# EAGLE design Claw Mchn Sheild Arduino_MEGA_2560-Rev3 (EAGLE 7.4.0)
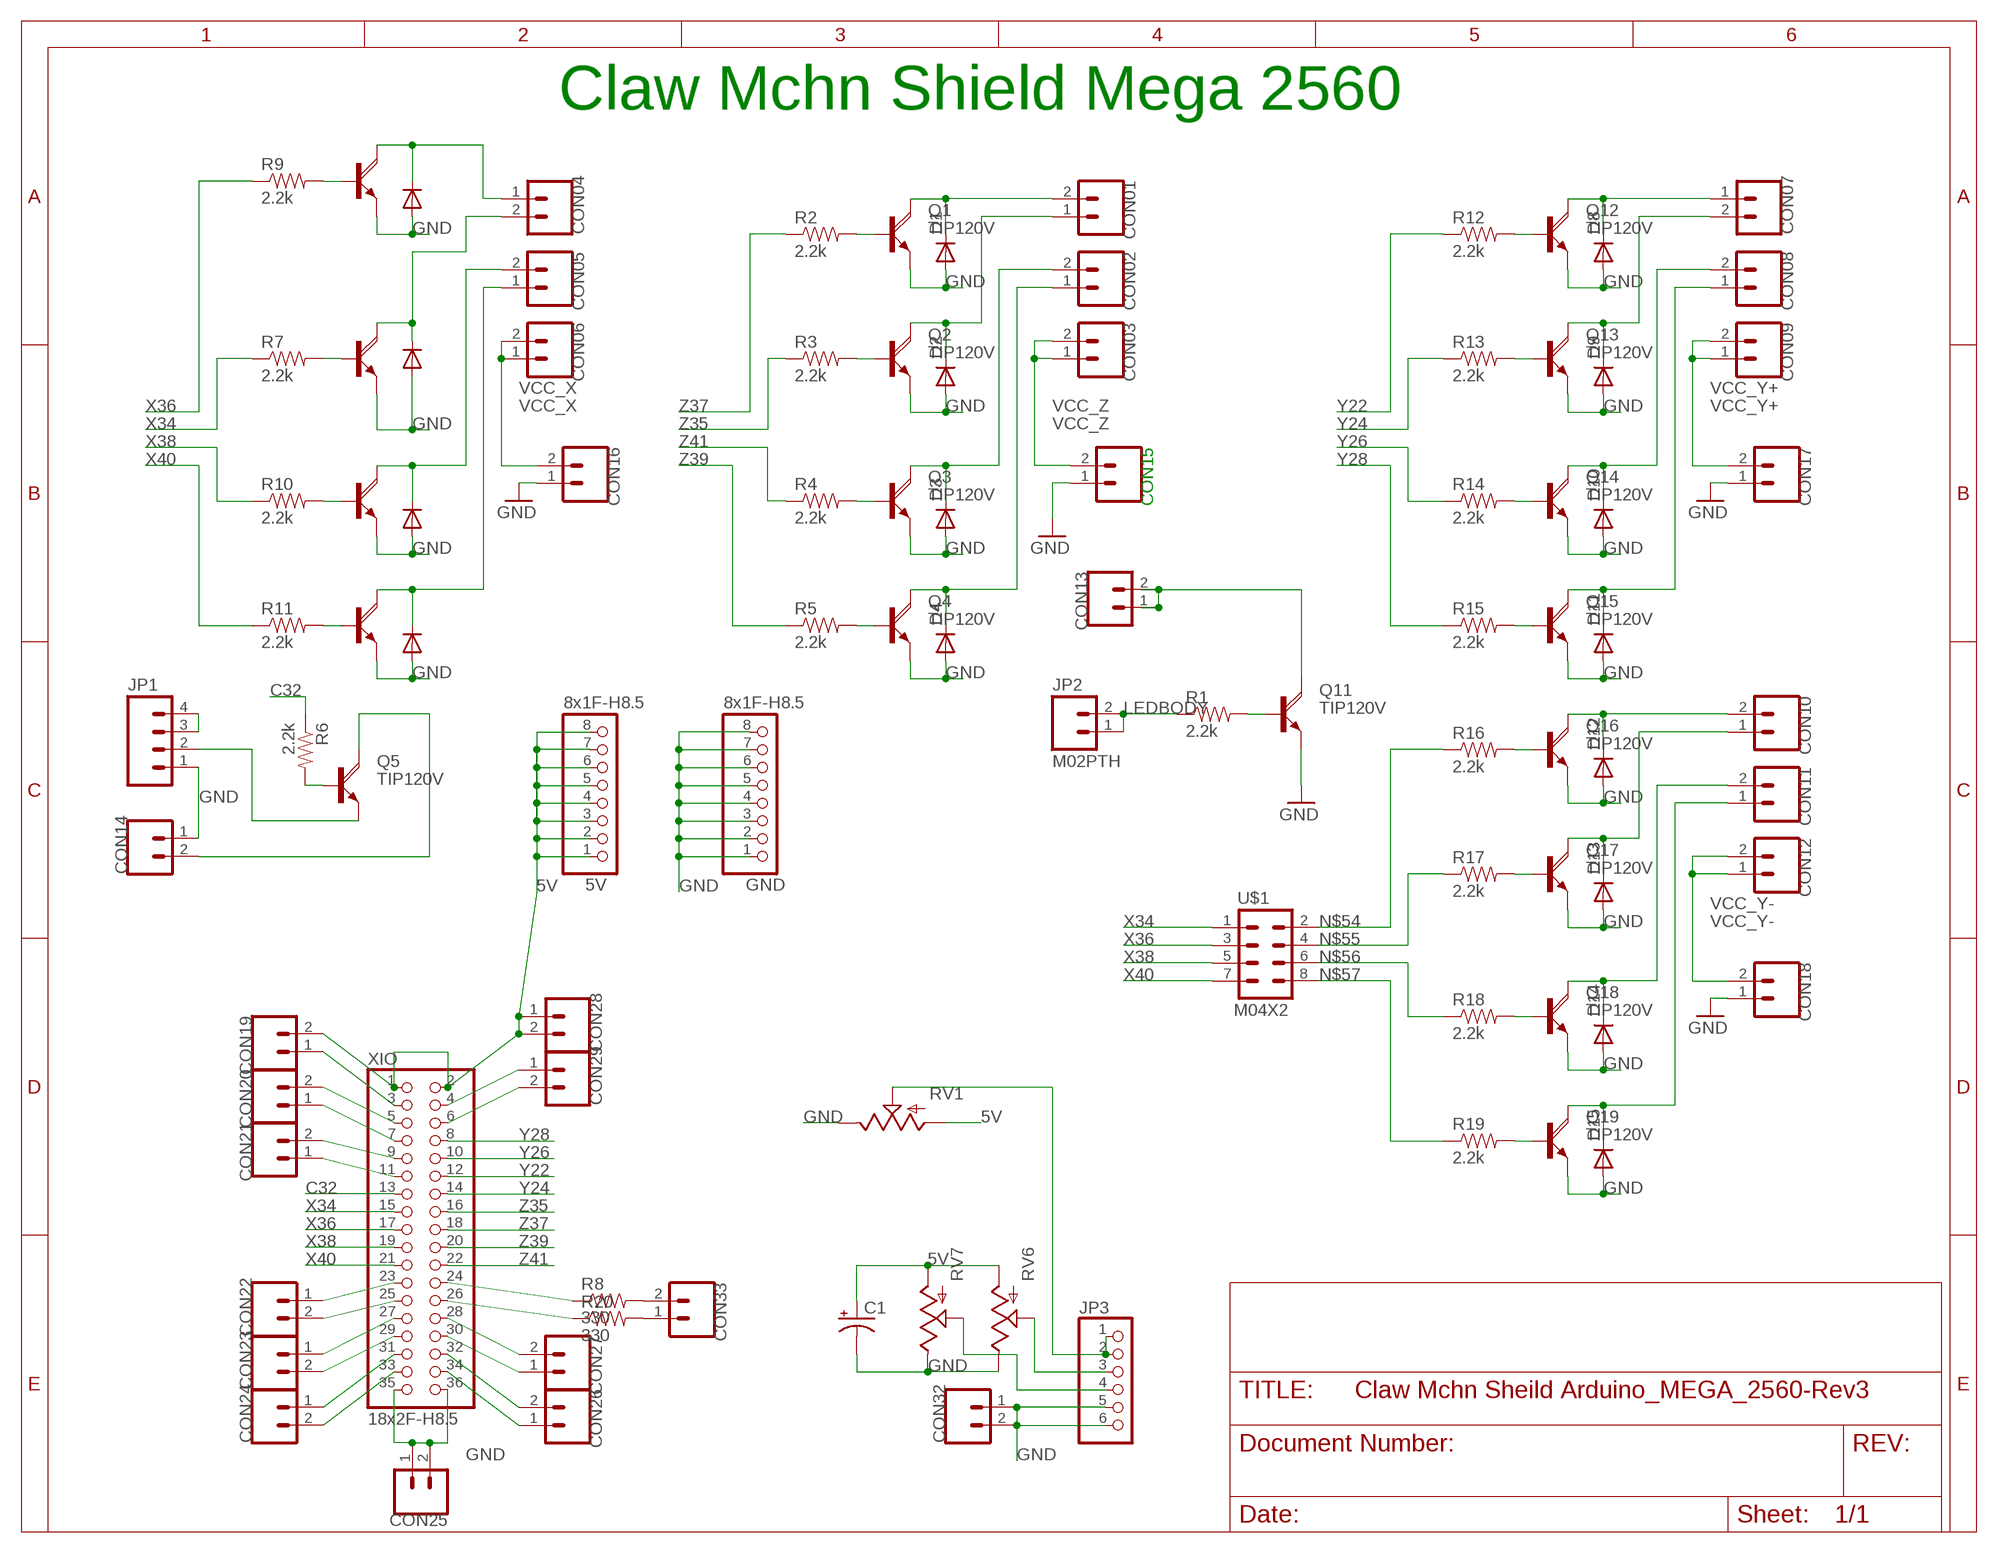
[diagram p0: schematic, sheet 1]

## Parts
5V  8x1F-H8.5  PINHD-1X8  [1X08]
C1  CAP_POLPTH1  [CPOL-RADIAL-100UF-25V]
CON01  M023.5MM  [SCREWTERMINAL-3.5MM-2]
CON02  M023.5MM  [SCREWTERMINAL-3.5MM-2]
CON03  M023.5MM  [SCREWTERMINAL-3.5MM-2]
CON04  M023.5MM  [SCREWTERMINAL-3.5MM-2]
CON05  M023.5MM  [SCREWTERMINAL-3.5MM-2]
CON06  M023.5MM  [SCREWTERMINAL-3.5MM-2]
CON07  M023.5MM  [SCREWTERMINAL-3.5MM-2]
CON08  M023.5MM  [SCREWTERMINAL-3.5MM-2]
CON09  M023.5MM  [SCREWTERMINAL-3.5MM-2]
CON10  M023.5MM  [SCREWTERMINAL-3.5MM-2]
CON11  M023.5MM  [SCREWTERMINAL-3.5MM-2]
CON12  M023.5MM  [SCREWTERMINAL-3.5MM-2]
CON13  M023.5MM  [SCREWTERMINAL-3.5MM-2]
CON14  M023.5MM  [SCREWTERMINAL-3.5MM-2]
CON15  M023.5MM  [SCREWTERMINAL-3.5MM-2]
CON16  M023.5MM  [SCREWTERMINAL-3.5MM-2]
CON17  M023.5MM  [SCREWTERMINAL-3.5MM-2]
CON18  M023.5MM  [SCREWTERMINAL-3.5MM-2]
CON19  M023.5MM  [SCREWTERMINAL-3.5MM-2]
CON20  M023.5MM  [SCREWTERMINAL-3.5MM-2]
CON21  M023.5MM  [SCREWTERMINAL-3.5MM-2]
CON22  M023.5MM  [SCREWTERMINAL-3.5MM-2]
CON23  M023.5MM  [SCREWTERMINAL-3.5MM-2]
CON24  M023.5MM  [SCREWTERMINAL-3.5MM-2]
CON25  M023.5MM  [SCREWTERMINAL-3.5MM-2]
CON26  M023.5MM  [SCREWTERMINAL-3.5MM-2]
CON27  M023.5MM  [SCREWTERMINAL-3.5MM-2]
CON28  M023.5MM  [SCREWTERMINAL-3.5MM-2]
CON29  M023.5MM  [SCREWTERMINAL-3.5MM-2]
CON32  M023.5MM  [SCREWTERMINAL-3.5MM-2]
CON33  M023.5MM  [SCREWTERMINAL-3.5MM-2]
D1  DIODE-SOT54H  [SOT54H]
D2  DIODE-SOT54H  [SOT54H]
D3  DIODE-SOT54H  [SOT54H]
D4  DIODE-SOT54H  [SOT54H]
D5  DIODE-SOT54H  [SOT54H]
D6  DIODE-SOT54H  [SOT54H]
D7  DIODE-SOT54H  [SOT54H]
D8  DIODE-SOT54H  [SOT54H]
D9  DIODE-SOT54H  [SOT54H]
D10  DIODE-SOT54H  [SOT54H]
D11  DIODE-SOT54H  [SOT54H]
D12  DIODE-SOT54H  [SOT54H]
D13  DIODE-SOT54H  [SOT54H]
D14  DIODE-SOT54H  [SOT54H]
D15  DIODE-SOT54H  [SOT54H]
D16  DIODE-SOT54H  [SOT54H]
GND  8x1F-H8.5  PINHD-1X8  [1X08]
JP1  M04PTH  [1X04]
JP2  M02PTH  [1X02]
JP3  PINHD-1X6  [1X06]
Q1  TIP120V  [TO220AV]
Q2  TIP120V  [TO220AV]
Q3  TIP120V  [TO220AV]
Q4  TIP120V  [TO220AV]
Q5  TIP120V  [TO220AV]
Q6  TIP120V  [TO220AV]
Q8  TIP120V  [TO220AV]
Q9  TIP120V  [TO220AV]
Q10  TIP120V  [TO220AV]
Q11  TIP120V  [TO220AV]
Q12  TIP120V  [TO220AV]
Q13  TIP120V  [TO220AV]
Q14  TIP120V  [TO220AV]
Q15  TIP120V  [TO220AV]
Q16  TIP120V  [TO220AV]
Q17  TIP120V  [TO220AV]
Q18  TIP120V  [TO220AV]
Q19  TIP120V  [TO220AV]
R1  2.2k  RESISTORPTH-1/6W  [1/6W-RES]
R2  2.2k  RESISTORPTH-1/6W  [1/6W-RES]
R3  2.2k  RESISTORPTH-1/6W  [1/6W-RES]
R4  2.2k  RESISTORPTH-1/6W  [1/6W-RES]
R5  2.2k  RESISTORPTH-1/6W  [1/6W-RES]
R6  2.2k  RESISTORPTH-1/6W  [1/6W-RES]
R7  2.2k  RESISTORPTH-1/6W  [1/6W-RES]
R8  330  RESISTORPTH-1/4W  [AXIAL-0.4]
R9  2.2k  RESISTORPTH-1/6W  [1/6W-RES]
R10  2.2k  RESISTORPTH-1/6W  [1/6W-RES]
R11  2.2k  RESISTORPTH-1/6W  [1/6W-RES]
R12  2.2k  RESISTORPTH-1/6W  [1/6W-RES]
R13  2.2k  RESISTORPTH-1/6W  [1/6W-RES]
R14  2.2k  RESISTORPTH-1/6W  [1/6W-RES]
R15  2.2k  RESISTORPTH-1/6W  [1/6W-RES]
R16  2.2k  RESISTORPTH-1/6W  [1/6W-RES]
R17  2.2k  RESISTORPTH-1/6W  [1/6W-RES]
R18  2.2k  RESISTORPTH-1/6W  [1/6W-RES]
R19  2.2k  RESISTORPTH-1/6W  [1/6W-RES]
R20  330  RESISTORPTH-1/4W  [AXIAL-0.4]
RV1  POTTRIM  [TRIM_POT]
RV6  POTTRIM  [TRIM_POT]
RV7  POTTRIM  [TRIM_POT]
U$1  M04X2  [2X4]
XIO  18x2F-H8.5  PINHD-2X18  [2X18]

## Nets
5V: 5V.1 5V.2 5V.3 5V.4 5V.5 5V.6 5V.7 5V.8 C1.1(+) CON19.2 CON28.1 CON28.2 RV1.3(A) RV6.3(A) RV7.3(A) XIO.1 XIO.2
C32: R6.1 XIO.13
GND: C1.2(-) CON14.1 CON15.1 CON16.1 CON17.1 CON18.1 CON25.1 CON25.2 CON32.1 CON32.2 D1.A D2.A D3.A D4.A D5.A D6.A D7.A D8.A D9.A D10.A D11.A D12.A D13.A D14.A D15.A D16.A GND.1 GND.2 GND.3 GND.4 GND.5 GND.6 GND.7 GND.8 JP1.1 JP3.5 JP3.6 Q1.E Q2.E Q3.E Q4.E Q6.E Q8.E Q9.E Q10.E Q11.E Q12.E Q13.E Q14.E Q15.E Q16.E Q17.E Q18.E Q19.E RV1.2(E) RV6.2(E) RV7.2(E) XIO.35 XIO.36
LEDBODY: JP2.1 JP2.2 R1.1
N$1: Q11.B R1.2
N$2: Q1.B R2.2
N$3: Q2.B R3.2
N$4: Q3.B R4.2
N$5: Q4.B R5.2
N$6: CON33.1 R20.P$2
N$7: CON04.2 D16.C Q6.C
N$8: CON26.1 XIO.34
N$9: CON27.1 XIO.30
N$10: CON01.2 D1.C Q1.C
N$11: CON01.1 D2.C Q2.C
N$12: CON02.2 D3.C Q3.C
N$13: CON02.1 D4.C Q4.C
N$14: CON21.1 XIO.11
N$15: CON33.2 R8.P$2
N$16: JP1.2 Q5.E
N$17: Q6.B R7.2
N$18: Q5.B R6.2
N$19: JP3.4 RV7.1(S)
N$21: CON29.1 XIO.4
N$22: R20.P$1 XIO.26
N$23: CON14.2 Q5.C
N$24: R8.P$1 XIO.24
N$25: Q8.B R9.2
N$26: Q9.B R10.2
N$27: Q10.B R11.2
N$28: CON21.2 XIO.9
N$29: CON26.2 XIO.32
N$30: CON27.2 XIO.28
N$31: CON20.1 XIO.7
N$32: CON20.2 XIO.5
N$33: CON04.1 D5.C Q8.C
N$34: CON05.2 D6.C Q9.C
N$35: CON05.1 D7.C Q10.C
N$36: Q12.B R12.2
N$37: CON24.2 XIO.33
N$38: Q13.B R13.2
N$39: CON13.1 CON13.2 Q11.C
N$40: Q14.B R14.2
N$41: Q15.B R15.2
N$42: CON24.1 XIO.31
N$43: CON23.2 XIO.29
N$44: CON23.1 XIO.27
N$45: CON22.2 XIO.25
N$46: CON07.1 D8.C Q12.C
N$47: CON07.2 D9.C Q13.C
N$48: CON08.2 D10.C Q14.C
N$49: CON08.1 D11.C Q15.C
N$50: Q16.B R16.2
N$51: Q17.B R17.2
N$52: Q18.B R18.2
N$53: Q19.B R19.2
N$54: R16.1 U$1.2
N$55: R17.1 U$1.4
N$56: R18.1 U$1.6
N$57: R19.1 U$1.8
N$58: CON10.2 D12.C Q16.C
N$59: CON10.1 D13.C Q17.C
N$60: CON11.2 D14.C Q18.C
N$61: CON11.1 D15.C Q19.C
N$62: CON19.1 XIO.3
N$63: CON22.1 XIO.23
N$65: JP1.3 JP1.4
N$66: CON29.2 XIO.6
N$67: JP3.3 RV6.1(S)
N$74: JP3.1 JP3.2 RV1.1(S)
VCC_X: CON06.1 CON06.2 CON16.2
VCC_Y+: CON09.1 CON09.2 CON17.2
VCC_Y-: CON12.1 CON12.2 CON18.2
VCC_Z: CON03.1 CON03.2 CON15.2
X34: R7.1 U$1.1 XIO.15
X36: R9.1 U$1.3 XIO.17
X38: R10.1 U$1.5 XIO.19
X40: R11.1 U$1.7 XIO.21
Y22: R12.1 XIO.12
Y24: R13.1 XIO.14
Y26: R14.1 XIO.10
Y28: R15.1 XIO.8
Z35: R3.1 XIO.16
Z37: R2.1 XIO.18
Z39: R5.1 XIO.20
Z41: R4.1 XIO.22

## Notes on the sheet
- Claw Mchn Shield Mega 2560

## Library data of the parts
5V GND = SmartPrj:PINHD-1X8: PIN HEADER
C1 = SparkFun-Capacitors:CAP_POL: Capacitor Polarized
CON01-CON09 CON10-CON29 CON32 CON33 JP2 = SparkFun-Connectors:M02: Standard 2-pin 0.1" header. Use with
D1-D16 = diode:DIODE-: DIODE
JP1 = SparkFun-Connectors:M04: Header 4 Standard 4-pin 0.1" header. Use with straight break away headers (SKU : PRT-00116), right angle break away headers (PRT-00553), swiss pins (PRT-00743), machine pins (PRT-00117), and female headers (PRT-00115). Molex polarized connector foot print use with SKU : PRT-08231 with associated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
JP3 = pinhead:PINHD-1X6: PIN HEADER
Q1-Q6 Q8-Q19 = rocketfarm:TIP120: NPN DARLINGTON TRANSISTOR
R1-R20 = SparkFun-Passives:RESISTOR: Resistor
RV1 RV6 RV7 = SparkFun-Electromechanical:POT
U$1 = SparkFun-Connectors:M04X2: .1" header, two rows of four.
XIO = SmartPrj:PINHD-2X18: PIN HEADER

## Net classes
1 power: width 0.61 mm, drill 0.406 mm, clearance 0.203 mm
2 gnd: width 0.305 mm, drill 0.406 mm, clearance 0.203 mm
3 power usb: width 0.508 mm, drill 0.406 mm, clearance 0.203 mm

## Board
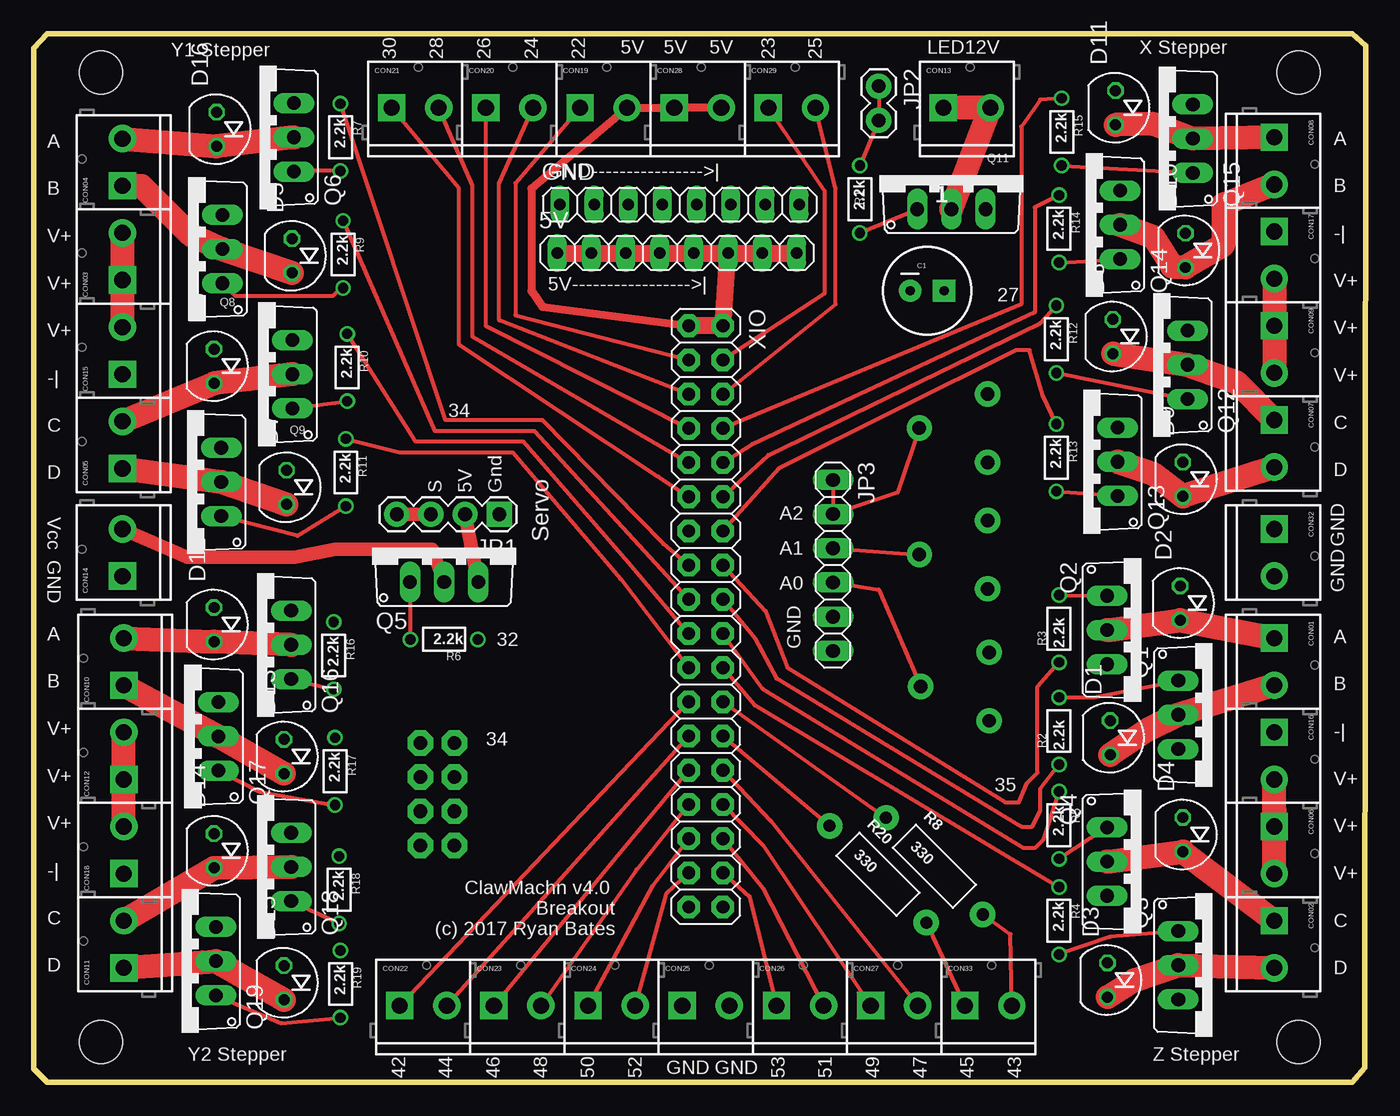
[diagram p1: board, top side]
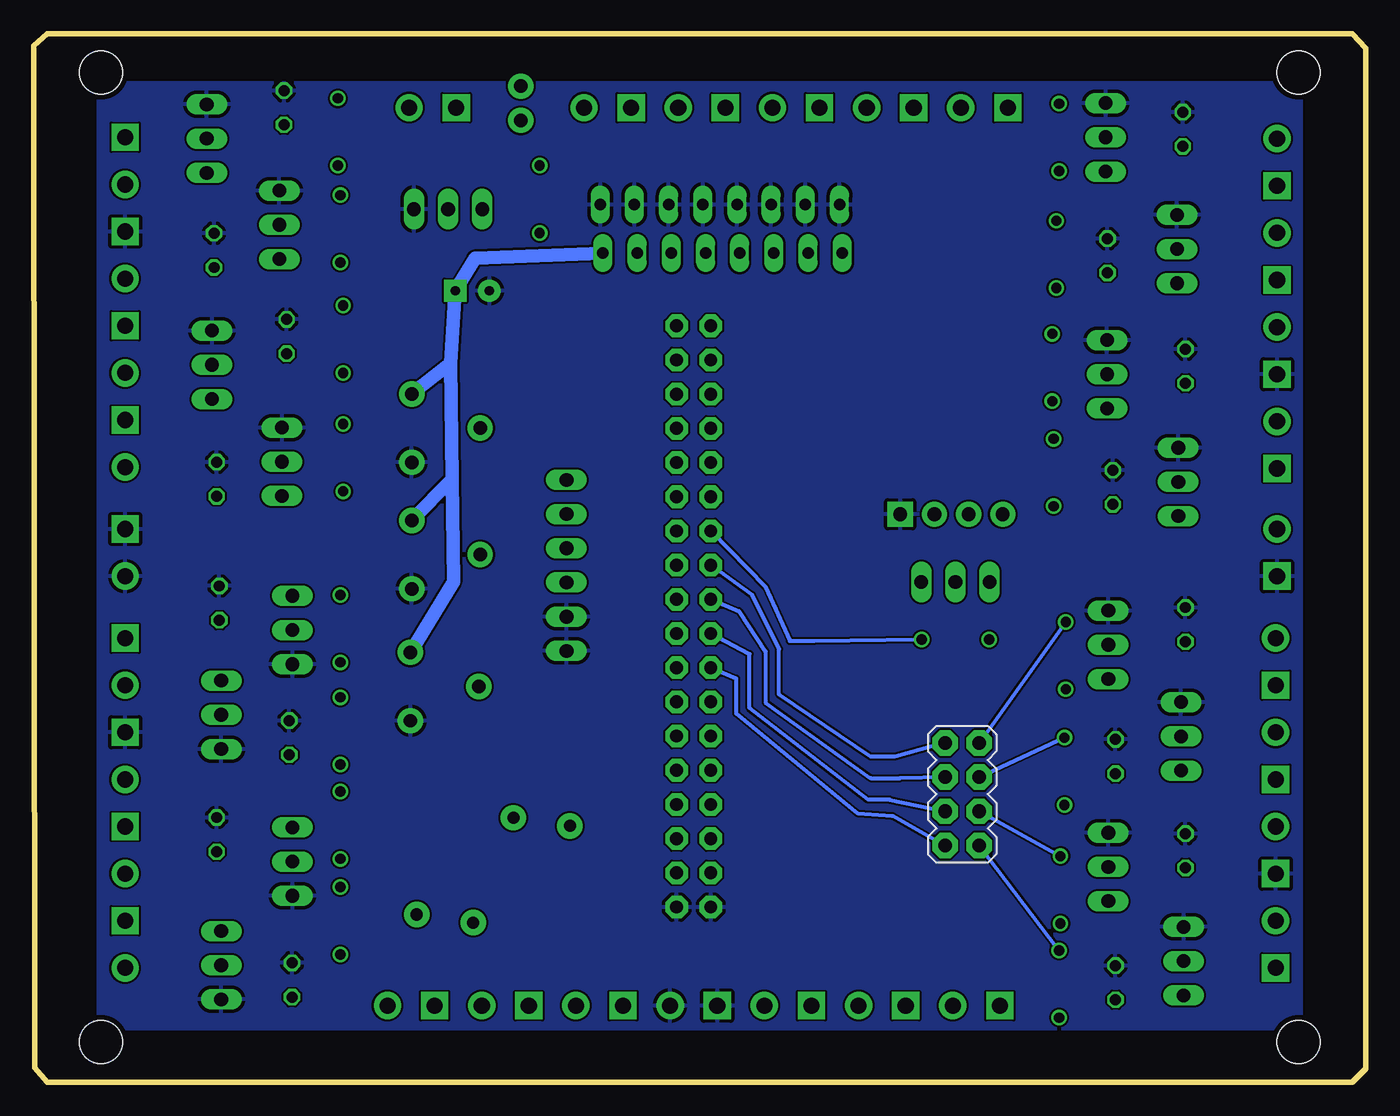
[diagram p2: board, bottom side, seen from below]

Size 99 x 77.9 mm. Coordinates in mm from the lower left corner, seen from the top.
Outline: 1,77.9 98,77.9 99,77 98.9,1.1 98,0 1,0 0,1 0,76.8 1,77.9
Copper layers (1*16): Top 0.0356mm / dielectric 1.5011mm / Bottom 0.0356mm
Design rules "OSHparkPCBOrder": minimum track width 6mil, minimum drill 13mil, track to track 6mil, track to pad 6mil, pad to pad 6mil, via to via 6mil, smd to smd 6mil, copper to edge 15mil, drill to drill 6mil, minimum pad ring 7mil, minimum via ring 7mil, stop-mask expansion 3mil, vias tented up to drill 0mil, thermal gap 10mil
Holes 3.2 mm at 94,3 5,75 94,75 5,3

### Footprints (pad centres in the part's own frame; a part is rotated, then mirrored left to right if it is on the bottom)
1X08 = drill 0.85 pad 1.422 long: 1 -8.89,0; 2 -6.35,0; 3 -3.81,0; 4 -1.27,0; 5 1.27,0; 6 3.81,0; 7 6.35,0; 8 8.89,0
CPOL-RADIAL-100UF-25V = drill 0.7 pad 1.651 square: 1 1.27,0 | drill 0.7 pad 1.651: 2 -1.27,0
SCREWTERMINAL-3.5MM-2 = drill 1.2 pad 2.032 square: 1 0,0 | drill 1.2 pad 2.032: 2 3.5,0
SOT54H = drill 0.813 octagon: A 1.27,0; C -1.27,0
1X04 = drill 1.016 pad 1.88 square: 1 0,0 | drill 1.016 pad 1.88: 2 2.54,0; 3 5.08,0; 4 7.62,0
1X02 = drill 1.016 pad 1.88: 1 0,0; 2 2.54,0
1X06 = drill 1.016 long: 1 -6.35,0; 2 -3.81,0; 3 -1.27,0; 4 1.27,0; 5 3.81,0; 6 6.35,0
TO220AV = drill 1.016 long: B -2.54,-2.54; C 0,-2.54; E 2.54,-2.54
1/6W-RES = drill 0.762: 1 -2.5,0; 2 2.5,0
AXIAL-0.4 = drill 0.9 pad 1.88: P$1 -5.08,0; P$2 5.08,0
TRIM_POT = drill 1 pad 1.88: 1 5.08,0; 2 0,2.54; 3 0,-2.54
2X4 = drill 1.016 pad 1.88 octagon: 1 -3.81,-1.27; 2 -3.81,1.27; 3 -1.27,-1.27; 4 -1.27,1.27; 5 1.27,-1.27; 6 1.27,1.27; 7 3.81,-1.27; 8 3.81,1.27
2X18 = drill 0.95 pad 1.676 octagon: 1 -21.59,-1.27; 2 -21.59,1.27; 3 -19.05,-1.27; 4 -19.05,1.27; 5 -16.51,-1.27; 6 -16.51,1.27; 7 -13.97,-1.27; 8 -13.97,1.27; 9 -11.43,-1.27; 10 -11.43,1.27; 11 -8.89,-1.27; 12 -8.89,1.27; 13 -6.35,-1.27; 14 -6.35,1.27; 15 -3.81,-1.27; 16 -3.81,1.27; 17 -1.27,-1.27; 18 -1.27,1.27; 19 1.27,-1.27; 20 1.27,1.27; 21 3.81,-1.27; 22 3.81,1.27; 23 6.35,-1.27; 24 6.35,1.27; 25 8.89,-1.27; 26 8.89,1.27; 27 11.43,-1.27; 28 11.43,1.27; 29 13.97,-1.27; 30 13.97,1.27; 31 16.51,-1.27; 32 16.51,1.27; 33 19.05,-1.27; 34 19.05,1.27; 35 21.59,-1.27; 36 21.59,1.27

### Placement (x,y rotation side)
5V  47.8,61.6 0 top
C1  66.4,58.8 0 top
CON01  92.2,33 270 top
CON02  92.2,12 270 top
CON03  6.6,59.6 90 top
CON04  6.6,66.6 90 top
CON05  6.6,45.6 90 top
CON06  92.2,19 270 top
CON07  92.2,49.2 270 top
CON08  92.2,70.2 270 top
CON09  92.2,56.2 270 top
CON10  6.7,29.5 90 top
CON11  6.7,8.5 90 top
CON12  6.7,22.5 90 top
CON13  67.6,72.4 0 top
CON14  6.6,37.6 90 top
CON15  6.6,52.6 90 top
CON16  92.2,26 270 top
CON17  92.2,63.2 270 top
CON18  6.7,15.5 90 top
CON19  40.6,72.4 0 top
CON20  33.6,72.4 0 top
CON21  26.6,72.4 0 top
CON22  27.2,5.7 0 top
CON23  34.2,5.7 0 top
CON24  41.2,5.7 0 top
CON25  48.2,5.7 0 top
CON26  55.2,5.7 0 top
CON27  62.2,5.7 0 top
CON28  47.6,72.4 0 top
CON29  54.6,72.4 0 top
CON32  92.2,41.1 270 top
CON33  69.2,5.7 0 top
D1  80,25.6 90 top
D2  85.2,35.6 90 top
D3  79.8,7.6 90 top
D4  85.4,18.4 90 top
D5  19.2,61.4 90 top
D6  13.4,53.2 90 top
D7  18.8,44.2 90 top
D8  80.2,55.4 90 top
D9  85.4,44.8 90 top
D10  85.6,61.8 90 top
D11  80.4,72.4 90 top
D12  13.4,34 90 top
D13  18.6,24.2 90 top
D14  13.4,17.2 90 top
D15  18.6,7.4 90 top
D16  13.6,70.8 90 top
GND  48,65.2 0 top
JP1  34.6,42.2 180 top
JP2  62.8,74 270 top
JP3  59.4,38.4 270 top
Q1  87.6,27.3 270 top
Q2  82.3,33.6 270 top
Q3  87.6,8.7 270 top
Q4  82.3,16.4 270 top
Q5  30.5,39.7 0 top
Q6  16.8,70.2 90 top
Q8  11.5,61.9 90 top
Q9  16.7,52.6 90 top
Q10  11.4,44.6 90 top
Q11  68.2,67.4 0 top
Q12  83.2,53.3 90 top
Q13  78,46.1 90 top
Q14  78.2,63.7 90 top
Q15  83.6,70.1 90 top
Q16  16.6,32.5 90 top
Q17  11.2,25.7 90 top
Q18  16.6,16 90 top
Q19  11,9 90 top
R1  61.4,65.6 270 top
R2  76.2,26.1 90 top
R3  76.2,33.7 90 top
R4  76.2,12 270 top
R5  76.2,19.1 270 top
R6  30.5,32.9 180 top
R7  22.8,70.2 270 top
R8  66.94,16.06 315 top
R9  23,61.5 270 top
R10  23.3,53.1 270 top
R11  23.2,45.3 270 top
R12  76,55.2 270 top
R13  76,46.4 270 top
R14  76.2,63.4 270 top
R15  76.4,70.6 270 top
R16  22.3,31.7 270 top
R17  22.4,23.1 270 top
R18  22.7,14.3 270 top
R19  22.8,7.3 270 top
R20  62.74,15.46 315 top
RV1  70.9,48.6 180 top
RV6  70.9,39.2 180 top
RV7  71,29.4 180 top
U$1  30,21.4 270 bottom
XIO  49.95,34.61 270 top

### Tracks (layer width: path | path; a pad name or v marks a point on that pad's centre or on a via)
5V
  Top 0.61: CON28.2 CON28.1 CON19.2 37,66.4 37,58.8 37.8,57.6 XIO.1
  Top 1.27: XIO.1 XIO.2 5V.6 | 5V.1 5V.2 5V.3 5V.4 5V.5 5V.6 | 5V.6 5V.7 5V.8
  Bottom 1.016: 5V.8 66.2,61.2 C1.1 68.01,53.4 | 68.01,53.4 67.9,44.81 | 67.9,44.81 67.8,37.2 RV7.3 | RV6.3 67.9,44.81 | RV1.3 68.01,53.4
C32
  Bottom 0.305: XIO.13 44.6,36.8 42.8,32.8 41,32.8 R6.1
GND
  pour Bottom: 4.8,74.2 94.2,74.2 94.2,4 4.8,4
LEDBODY
  Top 0.305: JP2.1 JP2.2 R1.1
N$1
  Top 0.305: R1.2 Q11.B
N$2
  Top 0.305: R2.2 78.8,28.6 Q1.B
N$3
  Top 0.305: R3.2 Q2.B
N$4
  Top 0.305: Q3.B 80,10.8 R4.2
N$5
  Top 0.305: R5.2 Q4.B
N$6
  Top 0.305: R20.P$2 CON33.1
N$7
  Top 1.778: CON04.2 D16.C Q6.C
N$8
  Top 0.305: XIO.34 53.2,13.8 CON26.1
N$9
  Top 0.305: XIO.30 54.2,17.6 CON27.1
N$10
  Top 1.778: CON01.2 Q1.C 82.8,26.2 D1.C
N$11
  Top 1.778: Q2.C D2.C CON01.1
N$12
  Top 1.778: CON02.2 Q3.C 81.8,7.6 D3.C
N$13
  Top 1.778: Q4.C D4.C CON02.1
N$14
  Top 0.305: XIO.11 46.4,45 31.6,54.8 31.6,66.4 CON21.1
N$15
  Top 0.305: CON33.2 72.6,11 R8.P$2
N$16
  Top 1.016: JP1.2 Q5.E
N$17
  Top 0.305: R7.2 19.38,67.7 Q6.B
N$18
  Top 0.305: R6.2 28,34.4 Q5.B
N$19
  Top 0.305: JP3.4 62.8,36.6 RV7.1
N$21
  Top 0.305: XIO.4 58.8,58.6 58.8,66.2 CON29.1
N$22
  Top 0.305: R20.P$1 XIO.26
N$23
  Top 1.016: Q5.C 29.6,39.6 22.4,39.6 19.4,39 11.4,39 CON14.2
N$24
  Top 0.305: XIO.24 R8.P$1
N$25
  Top 0.305: R9.2 22.8,59 22.2,58.4 15,58.4 Q8.B
N$26
  Top 0.305: Q9.B R10.2
N$27
  Top 0.305: R11.2 19.6,40.6 Q10.B
N$28
  Top 0.305: XIO.9 32.6,55.4 32.6,66.6 CON21.2
N$29
  Top 0.305: XIO.32 54.2,14.4 CON26.2
N$30
  Top 0.305: XIO.28 54.8,19.4 CON27.2
N$31
  Top 0.305: CON20.1 33.6,56.2 XIO.7
N$32
  Top 0.305: XIO.5 34.6,56.6 34.6,66.8 CON20.2
N$33
  Top 1.778: CON04.1 8,66.6 11.6,63 Q8.C D5.C
N$34
  Top 1.778: Q9.C D6.C CON05.2
N$35
  Top 1.778: CON05.1 Q10.C D7.C
N$36
  Top 0.305: R12.2 Q12.B
N$37
  Top 0.305: XIO.33 47,14 CON24.2
N$38
  Top 0.305: R13.2 Q13.B
N$39
  Top 1.778: Q11.C CON13.2 CON13.1
N$40
  Top 0.305: R14.2 Q14.B
N$41
  Top 0.305: R15.2 Q15.B
N$42
  Top 0.305: XIO.31 46,14.6 CON24.1
N$43
  Top 0.305: XIO.29 44.8,15.8 CON23.2
N$44
  Top 0.305: XIO.27 43.2,16.6 CON23.1
N$45
  Top 0.305: XIO.25 CON22.2
N$46
  Top 1.778: D8.C Q12.C 89.4,52 CON07.1
N$47
  Top 1.778: CON07.2 D9.C 83.2,45.2 Q13.C
N$48
  Top 1.778: Q14.C 83.2,62.8 84.6,60.6 D10.C 88.4,62.2 88.4,65.2 CON08.2
N$49
  Top 1.778: CON08.1 Q15.C 83.2,71.2 D11.C
N$50
  Top 0.305: Q16.B R16.2
N$51
  Top 0.305: Q17.B 16.8,21.6 R17.2
N$52
  Top 0.305: Q18.B R18.2
N$53
  Top 0.305: Q19.B 18.4,4.4 R19.2
N$54
  Bottom 0.305: R16.1 U$1.2
N$55
  Bottom 0.305: R17.1 U$1.4
N$56
  Bottom 0.305: R18.1 U$1.6
N$57
  Bottom 0.305: R19.1 U$1.8
N$58
  Top 1.778: CON10.2 D12.C Q16.C
N$59
  Top 1.778: CON10.1 Q17.C D13.C
N$60
  Top 1.778: CON11.2 D14.C Q18.C
N$61
  Top 1.778: CON11.1 Q19.C D15.C
N$62
  Top 0.305: CON19.1 35.8,66.8 35.8,57 XIO.3
N$63
  Top 0.305: XIO.23 CON22.1
N$65
  Top 1.016: JP1.4 JP1.3
N$66
  Top 0.305: XIO.6 59.6,57.8 59.6,66.4 CON29.2
N$67
  Top 0.305: JP3.3 RV6.1
N$74
  Top 0.305: RV1.1 64.2,43.8 JP3.2 JP3.1
VCC_X
  Top 1.778: CON16.2 92.2,20.2 CON06.1 CON06.2
VCC_Y+
  Top 1.778: CON17.2 CON09.1 CON09.2
VCC_Y-
  Top 1.778: CON18.2 CON12.1 CON12.2
VCC_Z
  Top 1.778: CON15.2 CON03.1 CON03.2
X34
  Top 0.305: XIO.15 46.8,40 37.8,49.2 30.6,49.2 R7.1
  Bottom 0.305: XIO.15 45.6,36.2 43.6,32.2 43.6,28.8 36.8,24.2 35,24.2 U$1.1
X36
  Top 0.305: R9.1 29.8,48.4 37.2,48.4 XIO.17
  Bottom 0.305: XIO.17 46.6,35 44.6,32 44.6,28.2 36.8,22.6 34.6,22.6 U$1.3
X38
  Top 0.305: XIO.19 44.2,38.6 36.4,47.6 28.4,47.6 R10.1
  Bottom 0.305: XIO.19 45.8,31.8 45.8,27.8 37,21 35.4,21 U$1.5
X40
  Top 0.305: R11.1 27.2,46.8 35.6,46.8 43.6,37.4 XIO.21
  Bottom 0.305: XIO.21 46.8,30 46.8,27.4 37.8,20 35.2,19.8 U$1.7
Y22
  Top 0.305: XIO.12 54.6,46.6 74.8,56.4 R12.1
Y24
  Top 0.305: R13.1 75,51 74,54.4 73,54.4 55.4,45.6 XIO.14
Y26
  Top 0.305: R14.1 74.4,65 74.4,57.2 53.4,47.4 XIO.10
Y28
  Top 0.305: R15.1 74.8,73 73.4,71 73.4,57.8 XIO.8
Z35
  Top 0.305: XIO.16 54.4,35 56,30.8 72.2,20.8 73.2,20.8 73.8,22.2 74.6,23 74.6,29.4 R3.1
Z37
  Top 0.305: XIO.18 53.6,33 55.2,30 73.4,19 74.2,19 74.8,20.2 74.8,21.8 R2.1
Z39
  Top 0.305: R5.1 75,18 74.4,17.4 73.6,17.4 54.2,29.2 XIO.20
Z41
  Top 0.305: R4.1 53.6,28 XIO.22

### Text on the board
tPlace: X Stepper | Y1 Stepper | 30 / / 28 / / 26 / / 24 / / 22 | 5V | 5V | 5V | 23 / / 25 | LED12V | GND---------------->| | 5V----------------->| | 27 | 34 | A / / B / / V+ / / V+ / / V+ / / -| / / C / / D | Servo | A / / B / / -| / / V+ / / V+ / / V+ / / C / / D | S / 5V / Gnd | A2 | Vcc | A1 | GND | GND | A0 | GND | 32 | GND | 34 | 35 | ClawMachn v4.0 / Breakout / (c) 2017 Ryan Bates | A / / B / / V+ / / V+ / / V+ / / -| / / C / / D | A / / B / / -| / / V+ / / V+ / / V+ / / C / / D | Y2 Stepper | Z Stepper | GND | GND | 42 / / 44 / / 46 / / 48 / / 50 / / 52 | 53 / / 51 / / 49 / / 47 / / 45 / / 43
tNames: 1

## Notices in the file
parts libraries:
SparkFun-Aesthetics: Licensing: Creative Commons ShareAlike 4.0 International - https://creativecommons.org/licenses/by-sa/4.0
